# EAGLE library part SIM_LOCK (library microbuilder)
C707A SIMLOCK® 2.5 mm with wide solder tails Source: Data sheet
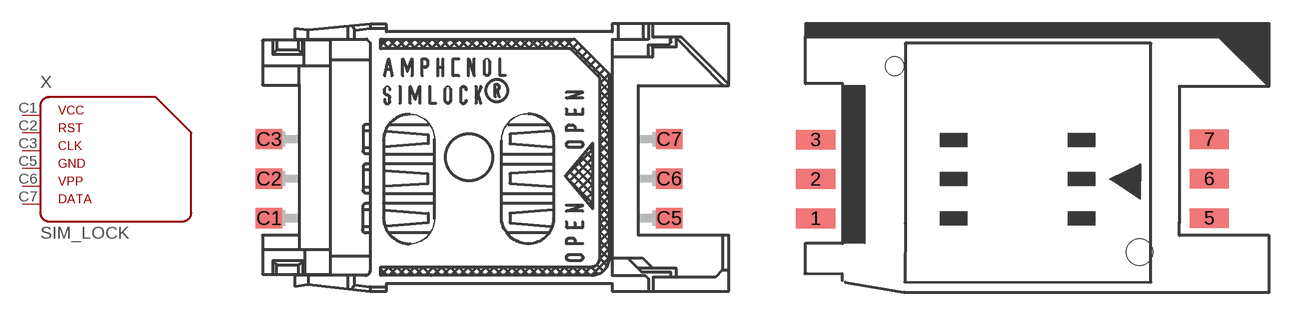
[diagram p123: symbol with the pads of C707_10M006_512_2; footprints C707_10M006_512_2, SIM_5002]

Designator prefix X

## SIM_LOCKAMPHENOL (OC_FARNELL: unknown; OC_NEWARK: unknown)  [C707_10M006_512_2]
C1  1  pas
C2  2  pas
C3  3  pas
C5  4  pas
C6  5  pas
C7  6  pas

## SIM_LOCK  [SIM_5002]
1  1  pas
2  2  pas
3  3  pas
5  4  pas
6  5  pas
7  6  pas

## Footprint C707_10M006_512_2 (pad centres in mm)
C707A SIMLOCK® 2.5 mm with wide solder tails Source: Data sheet
smd 1.7 x 1.3: C1 -12.85,-3.915; C2 -12.85,-1.375; C3 -12.85,1.165; C5 12.85,-3.915; C6 12.85,-1.375; C7 12.85,1.165

## Footprint SIM_5002 (pad centres in mm)
6 Contacts (3+3), low profile drawn by DeSIG desig@radikaldesig.com
smd 2.54 x 1.27: 1 0.904,0.574; 2 0.904,3.114; 3 0.904,5.654; 5 26.299,0.594; 6 26.299,3.134; 7 26.299,5.674
hole 1.7 at 21.8,-1.6
hole 1.2 at 6,10.4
